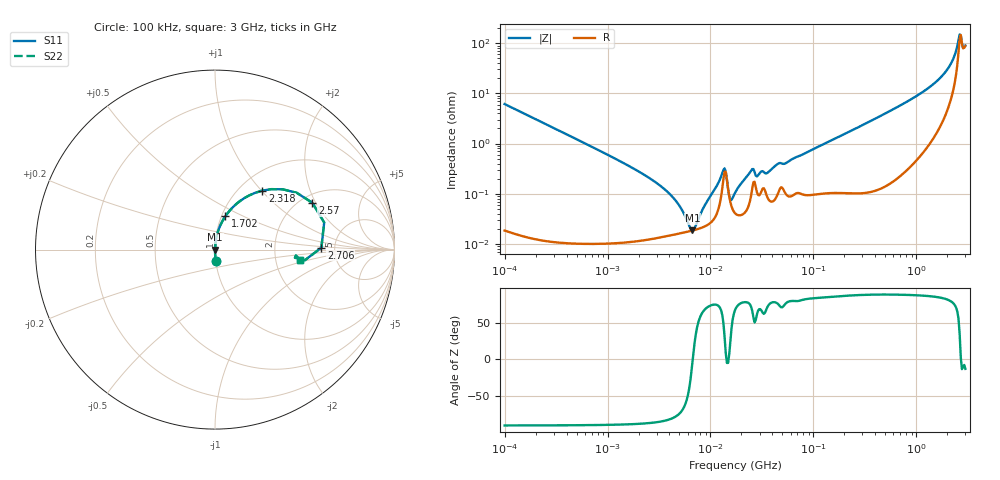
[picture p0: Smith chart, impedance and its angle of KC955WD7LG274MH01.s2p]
!Murata Part Number: KC955WD7LG274MH01
!These Parameters are Measured in Series Mode Connection
!Data Generated on Mar 13, 2026
!  o--ll--o
!Port1  Port2
!  o------o
!Operation Temp=25[degC], DC Bias Voltage=0[V]
!Freq. Start=100[kHz] Stop=3[GHz] 401[Steps]
# Hz S RI R 50
!Freq.(Hz) S11(Real) S11(Imag) S21(Real) S21(Imag) S12(Real) S12(Imag) S22(Real) S22(Imag)
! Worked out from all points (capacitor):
!   401 points, 100 kHz to 3 GHz, reference 50 ohm
!   read as one part in series: C = 259 nF near 105.3 kHz
!   lowest |Z| = 18.6 mohm at 6.675 MHz (marker M1)
!   series resonance near 6.729 MHz, so ESL is about 2.2 nH
!   S11 on the Smith chart (normalised r, x): 100 kHz: 1.00, -0.12; 1.702 GHz: 1.04, +0.40; 2.318 GHz: 1.27, +1.01; 2.57 GHz: 2.30, +1.88; 2.706 GHz: 3.91, +0.13; 3 GHz: 2.76, -0.41
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100000  0.00394 -0.0611  0.9961 0.0611  0.9961 0.0611  0.00394 -0.0611
562235  0.000218 -0.0108  0.9998 0.0108  0.9998 0.0108  0.000218 -0.0108
3161081  0.000135 -0.00151  0.9999 0.00151  0.9999 0.00151  0.000135 -0.00151
4652942  0.000157 -0.000689  0.9998 0.000689  0.9998 0.000689  0.000157 -0.000689
6674626  0.000185 -1.5e-05  0.9998 1.5e-05  0.9998 1.5e-05  0.000185 -1.5e-05
1.338544e7  0.002 0.00224  0.998 -0.00224  0.998 -0.00224  0.002 0.00224
1.409348e7  0.0027 0.000374  0.9973 -0.000374  0.9973 -0.000374  0.0027 0.000374
1.56239e7  0.000678 0.000321  0.9993 -0.000321  0.9993 -0.000321  0.000678 0.000321
1.645034e7  0.000486 0.000676  0.9995 -0.000676  0.9995 -0.000676  0.000486 0.000676
1.77727e7  0.000392 0.00108  0.9996 -0.00108  0.9996 -0.00108  0.000392 0.00108
2.484619e7  0.000931 0.00274  0.9991 -0.00274  0.9991 -0.00274  0.000931 0.00274
2.826337e7  0.00108 0.00193  0.9989 -0.00193  0.9989 -0.00193  0.00108 0.00193
3.564176e7  0.000866 0.00244  0.9991 -0.00244  0.9991 -0.00244  0.000866 0.00244
4.494634e7  0.000986 0.0038  0.999 -0.0038  0.999 -0.0038  0.000986 0.0038
9.738194e7  0.001 0.00748  0.999 -0.00748  0.999 -0.00748  0.001 0.00748
5.475153e8  0.00348 0.0437  0.9965 -0.0437  0.9965 -0.0437  0.00348 0.0437
1.701687e9  0.0576 0.1854  0.9424 -0.1854  0.9424 -0.1854  0.0576 0.1854
2.038117e9  0.1257 0.2599  0.8743 -0.2599  0.8743 -0.2599  0.1257 0.2599
2.318426e9  0.2641 0.3287  0.7359 -0.3287  0.7359 -0.3287  0.2641 0.3287
2.570185e9  0.5425 0.2608  0.4575 -0.2608  0.4575 -0.2608  0.5425 0.2608
2.706139e9  0.5927 0.0108  0.4073 -0.0108  0.4073 -0.0108  0.5927 0.0108
3e9  0.4742 -0.0567  0.5258 0.0567  0.5258 0.0567  0.4742 -0.0567
